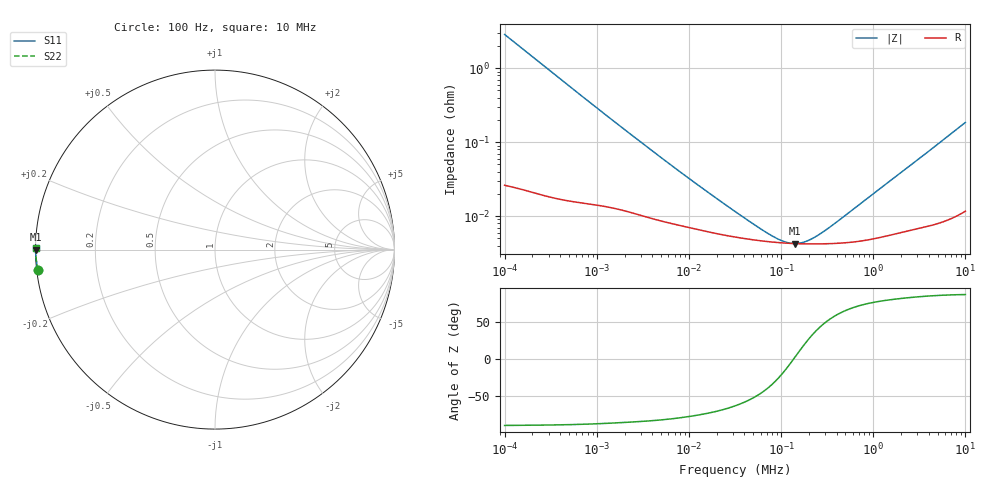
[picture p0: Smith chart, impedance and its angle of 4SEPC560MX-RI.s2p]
!  *** S-Parameter ***
!  Copyright (C) Panasonic Industry
!  Conductive Polymer Aluminum Solid Capacitors (OS-CON)
!  Parts No. 4SEPC560MX
! Touchstone file from project
# GHZ S RI R 50.000000
! Modal data exported
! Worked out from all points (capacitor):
!   401 points, 100 Hz to 10 MHz, reference 50 ohm
!   read as one part in shunt: C = 556 uF near 105.9 Hz
!   lowest |Z| = 4.26 mohm at 141.3 kHz (marker M1)
!   series resonance near 137.2 kHz, so ESL is about 2.4 nH
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1e-07  -0.9861 -0.1127  0.0139 -0.1127  0.0139 -0.1127  -0.9861 -0.1127
! Port Impedance 5.000000E+001 0.000000E+000 5.000000E+001 0.000000E+000
1.059254e-07  -0.9875 -0.1066  0.0125 -0.1066  0.0125 -0.1066  -0.9875 -0.1066
1.539927e-07  -0.9936 -0.0739  0.00641 -0.0739  0.00641 -0.0739  -0.9936 -0.0739
2.304093e-07  -0.9967 -0.0497  0.00327 -0.0497  0.00327 -0.0497  -0.9967 -0.0497
3.758374e-07  -0.9984 -0.0306  0.00162 -0.0306  0.00162 -0.0306  -0.9984 -0.0306
6.878599e-07  -0.9991 -0.0168  0.000884 -0.0168  0.000884 -0.0168  -0.9991 -0.0168
4.731513e-06  -0.9996 -0.00258  0.000356 -0.00258  0.000356 -0.00258  -0.9996 -0.00258
1.154782e-05  -0.9997 -0.0011  0.00027 -0.0011  0.00027 -0.0011  -0.9997 -0.0011
3.162278e-05  -0.9998 -0.000413  0.000209 -0.000413  0.000209 -0.000413  -0.9998 -0.000413
5.78762e-05  -0.9998 -0.000205  0.000187 -0.000205  0.000187 -0.000205  -0.9998 -0.000205
8.413951e-05  -0.9998 -0.000109  0.000177 -0.000109  0.000177 -0.000109  -0.9998 -0.000109
9.71628e-05  -0.9998 -7.62e-05  0.000175 -7.62e-05  0.000175 -7.62e-05  -0.9998 -7.62e-05
0.0001122018  -0.9998 -4.41e-05  0.000173 -4.41e-05  0.000173 -4.41e-05  -0.9998 -4.41e-05
0.0001258925  -0.9998 -1.88e-05  0.000171 -1.88e-05  0.000171 -1.88e-05  -0.9998 -1.88e-05
0.0001412538  -0.9998 6.4e-06  0.00017 6.4e-06  0.00017 6.4e-06  -0.9998 6.4e-06
0.0001727826  -0.9998 5.12e-05  0.000169 5.12e-05  0.000169 5.12e-05  -0.9998 5.12e-05
0.0002175204  -0.9998 0.000105  0.000168 0.000105  0.000168 0.000105  -0.9998 0.000105
0.0002660725  -0.9998 0.000157  0.000168 0.000157  0.000168 0.000157  -0.9998 0.000157
0.0003548134  -0.9998 0.000243  0.00017 0.000243  0.00017 0.000243  -0.9998 0.000243
0.001496236  -0.9998 0.00116  0.000221 0.00116  0.000221 0.00116  -0.9998 0.00116
0.009440609  -0.9995 0.00697  0.000495 0.00697  0.000495 0.00697  -0.9995 0.00697
0.01  -0.9995 0.00737  0.00052 0.00737  0.00052 0.00737  -0.9995 0.00737
